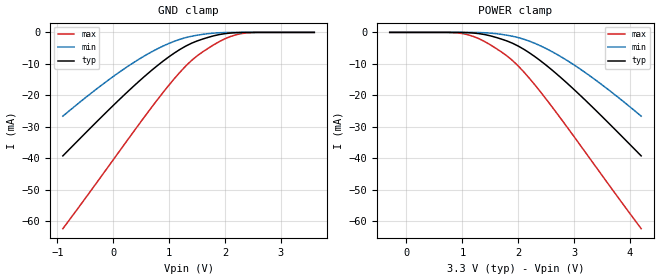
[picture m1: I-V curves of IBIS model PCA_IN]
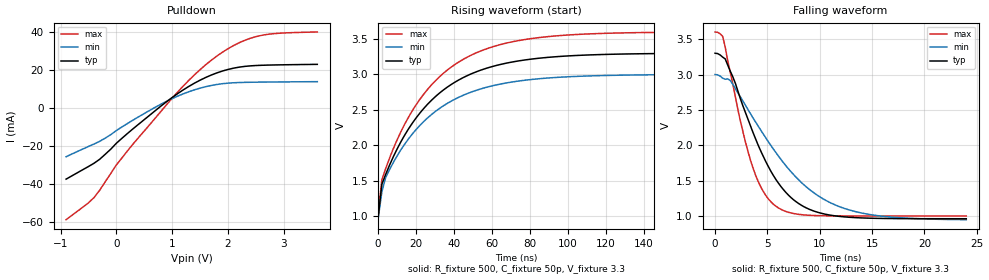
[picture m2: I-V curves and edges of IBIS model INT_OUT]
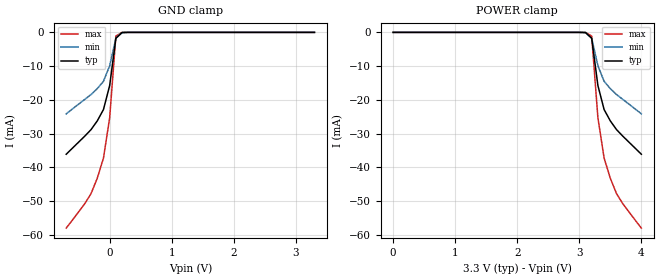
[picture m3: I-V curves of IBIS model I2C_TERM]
|  PCA9541 IBIS MODEL  by NXP Semiconductors, Specialty Logic, Tempe, AZ
|  2-to-1 I2C demultiplexer with interrupt logic and reset
|   Packages: SO16. TSSOP16, HVQFN16
[IBIS Ver]   3.2
[Comment Char]   |_char
| VDD Typ:3.3V, Min:3v, Max: 3.6v
[File name]   pca9541_3_3v.ibs
[File Rev]   1.0
[Date]   Apr 11, 2008 11:44:40 AM
[Source]
Generated by Seshadri Venkataramanan using IbisToolKit.
[Notes]
[Disclaimer]
(C) Copyright 2007 NXP Semiconductors
All rights reserved
NXP Semiconductors (NXP) does not warrant that this model and any other
accompanying information (Model) accurately or fully represents the
operating characteristics and specifications of the semiconductor
products to which the Model relates.  Moreover, the Model is furnished
on an "as is" and with "all faults" basis, and without support or
warranty of any kind.  NXP disclaims all warranties, whether expressed
or implied or statutory, including without limitation all implied
warranties of non-infringement, merchantability and fitness for any
purpose, and those arising from a course of dealing or usage of trade.
NXP does not convey any license under its or any third party's patents,
copyrights or other intellectual property or proprietary rights.
You and your company assume any and all risks and liability arising out
of the application or use of the Model.
In no event shall NXP be liable for any direct, indirect, special,
consequential or incidental damages, however caused, whether in
warranty, contract or tort (including negligence), strict liability or
other legal theory, including, without limitation, for lost profits,
business interruption, or corruption or loss of data or information,
arising out of or in connection with the use of or the inability to use
the Model, even if NXP has been advised of the possibility of such
damages.
NXP provides the Model as a courtesy to our customers. You and your
company shall not distribute, convey, sell, or give the Model to anyone
else without receiving prior written permission from NXP.
NXP reserves the right to make changes without notice to the Model to
improve reliability, function, or design.
Please be aware that your receipt and subsequent use of the Model shall
serve as acceptance of these terms and conditions.  If you do not
accept these terms, return or destroy the Model immediately.
[Copyright]
2008
[Component]   pca9541-1D
Si_location Pin
Timing_location Pin
[Manufacturer]   NXP Semiconductors
| [Package]   SO16
| [Package]   SO16
[Package]
|  variable   typ   min   max
R_pkg   1.75E-01   1.28E-01   2.11E-01
L_pkg   5.03E-09   3.94E-09   6.26E-09
C_pkg   0.794E-12   0.715E-12   0.869E-12
[Pin] signal_name   model_name   R_pin   L_pin   C_pin
1   INT0B   INT_OUT   1.99E-01  6.26E-09  0.822E-12
2   SDA_MST0   I2C_TERM   2.11E-01  5.46E-09  0.869E-12
3   SCL_MST0   I2C_TERM   1.56E-01  4.44E-09  0.760E-12
4   RESETB   PCA_IN   1.28E-01  3.94E-09  0.717E-12
5   SCL_MST1   I2C_TERM   1.28E-01  3.94E-09  0.715E-12
6   SDA_MST1   I2C_TERM   1.56E-01  4.44E-09  0.760E-12
7   INT1B   INT_OUT   2.11E-01  5.46E-09  0.869E-12
8   VSS   GND   1.99E-01  6.26E-09  0.843E-12
9   A0   PCA_IN   1.99E-01  6.26E-09  0.843E-12
10   A1   PCA_IN   2.11E-01  5.46E-09  0.869E-12
11   A2   PCA_IN   1.56E-01  4.44E-09  0.760E-12
12   A0(I2C_SEL)   PCA_IN   1.28E-01  3.94E-09  0.717E-12
13   SCL_SLAVE   I2C_TERM   1.28E-01  3.94E-09  0.715E-12
14   SDA_SLAVE   I2C_TERM   1.56E-01  4.44E-09  0.760E-12
15   INT_INB   PCA_IN   2.11E-01  5.46E-09  0.869E-12
16   VDD   POWER   1.99E-01  6.26E-09  0.843E-12
[Series Pin Mapping] pin_2 model_name   function_table_group
2   14   PCA_SW1   1
6   14   PCA_SW1   2
3   13   PCA_SW1   1
5   13   PCA_SW1   2
[Series Switch Groups]
|  1 /
On 1 /
|  2/
On 2 /
[Component]   pca9541-1PW
Si_location Pin
Timing_location Pin
[Manufacturer]   NXP Semiconductors
| [Package]   TSSOP16
| [Package]   TSSOP16
[Package]
| variable   typ   min   max
R_pkg   3.95E-02   3.52E-02   4.56E-02
L_pkg   1.94E-09   1.65E-09   2.40E-09
C_pkg   0.446E-12   0.335E-12   0.771E-12
[Pin] signal_name   model_name   R_pin   L_pin   C_pin
1   INT0B   INT_OUT   3.52E-02  2.40E-09  0.436E-12
2   SDA_MST0   I2C_TERM   3.70E-02  1.93E-09  0.438E-12
3   SCL_MST0   I2C_TERM   4.56E-02  1.76E-09  0.345E-12
4   RESETB   PCA_IN   4.00E-02  1.65E-09  0.335E-12
5   SCL_MST1   I2C_TERM   4.00E-02  1.65E-09  0.335E-12
6   SDA_MST1   I2C_TERM   4.56E-02  1.76E-09  0.345E-12
7   INT1B   INT_OUT   3.70E-02  1.93E-09  0.438E-12
8   VSS   GND   3.52E-02  2.40E-09  0.452E-12
9   A0   PCA_IN   3.52E-02  2.40E-09  0.452E-12
10   A1   PCA_IN   3.70E-02  1.93E-09  0.438E-12
11   A2   PCA_IN   4.56E-02  1.76E-09  0.345E-12
12   A0(I2C_SEL)   PCA_IN   4.00E-02  1.65E-09  0.771E-12
13   SCL_SLAVE   I2C_TERM   4.00E-02  1.65E-09  0.771E-12
14   SDA_SLAVE   I2C_TERM   4.56E-02  1.76E-09  0.345E-12
15   INT_INB   PCA_IN   3.70E-02  1.93E-09  0.438E-12
16   VDD   POWER   3.52E-02  2.40E-09  0.452E-12
[Series Pin Mapping] pin_2 model_name   function_table_group
2   14   PCA_SW1   1
6   14   PCA_SW1   2
3   13   PCA_SW1   1
5   13   PCA_SW1   2
[Series Switch Groups]
|  1 /
On 1 /
|  2/
On 2 /
[Component]   pca9541-1BS
Si_location Pin
Timing_location Pin
[Manufacturer]   NXP Semiconductors
[Package]
|  variable   typ   min   max
R_pkg   403m   325m   479m
L_pkg   112nh   98nh   127nh
C_pkg   0.142p   0.129p   0.157p
[Package Model]   hvqfn16
[Pin] signal_name   model_name
1   SCL_MST0   I2C_TERM
2   RESETB   PCA_IN
3   SCL_MST1   I2C_TERM
4   SDA_MST1   I2C_TERM
5   INT1B   INT_OUT
6   VSS   GND
7   A0   PCA_IN
8   A1   PCA_IN
9   A2   PCA_IN
10   A0(I2C_SEL)   PCA_IN
11   SCL_SLAVE   I2C_TERM
12   SDA_SLAVE   I2C_TERM
13   INT_INB   PCA_IN
14   VDD   POWER
15   INT0B   INT_OUT
16   SDA_MST0   I2C_TERM
[Series Pin Mapping] pin_2 model_name   function_table_group
16   12   PCA_SW1   1
4   12   PCA_SW1   2
1   11   PCA_SW1   1
3   11   PCA_SW1   2
[Series Switch Groups]
|  1 /
On 1 /
|  2/
On 2 /
[Define Package Model]   hvqfn16
[Manufacturer]   Unknown
[OEM]   Unknown
[Description]   none
[Number of Pins]   16
[Pin Numbers]
|   1 =
1
|   2 =
2
|   3 =
3
|   4 =
4
|   5 =
5
|   6 =
6
|   7 =
7
|   8 =
8
|   9 =
9
|   10 =
10
|   11 =
11
|   12 =
12
|   13 =
13
|   14 =
14
|   15 =
15
|   16 =
16
[Model Data]
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[End Model Data]
[End Package Model]
[Model]   PCA_SW1
Model_type Series_switch
C_comp   5.5p   5.3p   5.7p
[Temperature Range] 27   85   -40
[Voltage Range]   3.3   3   3.6
[On]
[R Series]   12   4   24
[L Series]   0   0   0
[C Series]   2p   1p   5p
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[Off]
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| Models and submodels in the file (4): PCA_IN (Input), INT_OUT (Open_drain), I2C_TERM (Terminator), PCA_SW1 (Series_switch)
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[Model]   PCA_IN
Model_type Input
Vinh=2.1
Vinl=0.9
C_comp   2.44p   2.2p   2.6p
[Temperature Range] 27   85   -40
[Voltage Range]   3.3   3   3.6
[GND Clamp]
-900mV    -39.22mA   -26.6mA    -62.33mA
-100mV    -24.97mA   -15.33mA   -42.96mA
500mV     -14.94mA   -8.108mA   -28.28mA
800mV     -10.43mA   -5.142mA   -21.2mA
1.1V      -6.496mA   -2.786mA   -14.59mA
1.3V      -4.347mA   -1.651mA   -10.68mA
1.5V      -2.735mA   -904.6uA   -7.49mA
1.9V      -688.8uA   -114uA     -2.915mA
2.1V      -205uA     -16.81uA   -1.301mA
2.3V      -30.06uA   -1.317uA   -370uA
2.6V      -376.8nA   -17.96nA   -10.03uA
3.6V      11.35pA    121.4pA    -358.3fA
[POWER Clamp]
-300mV    11.35pA    121.4pA    -358.3fA
700mV     -376.8nA   -17.96nA   -10.03uA
1V        -30.06uA   -1.317uA   -370uA
1.2V      -205uA     -16.81uA   -1.301mA
1.4V      -688.8uA   -114uA     -2.915mA
1.8V      -2.735mA   -904.6uA   -7.49mA
2V        -4.347mA   -1.651mA   -10.68mA
2.2V      -6.496mA   -2.786mA   -14.59mA
2.5V      -10.43mA   -5.142mA   -21.2mA
2.8V      -14.94mA   -8.108mA   -28.28mA
3.4V      -24.97mA   -15.33mA   -42.96mA
4.2V      -39.22mA   -26.6mA    -62.33mA
[Model]   INT_OUT
Model_type Open_drain
Vref=3.3
Vmeas=1.65
Rref=1000
Cref=50p
C_comp   2.44p   2.2p   2.6p
[Model Spec]
Vmeas   1.65   1.485   1.815
[Temperature Range] 27   85   -40
[Voltage Range]   3.3   3   3.6
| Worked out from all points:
|   slope of the pulldown table from 0 to 0.495 V, typ, clamps not added: 40.1 ohm
|   falling waveform, R_fixture 500, C_fixture 50p, V_fixture 3.3: 20-80 % time 4.2ns typ, 6.36ns min, 2.65ns max; typ from 3.3 V to 0.966 V
|   rising waveform, R_fixture 500, C_fixture 50p, V_fixture 3.3: 20-80 % time 35.2ns typ, 34.2ns min, 35.2ns max; typ from 0.966 V to 3.3 V
[Pulldown]
-900mV    -37.63mA   -25.83mA   -59mA
-400mV    -29.27mA   -19.11mA   -47.35mA
-300mV    -27.2mA    -17.72mA   -43.56mA
0V        -18.73mA   -12.01mA   -30.14mA
600mV     -3.874mA   -1.355mA   -8.841mA
1V        5.408mA    4.822mA    5.042mA
1.4V      12.97mA    9.452mA    17.37mA
1.8V      18.37mA    12.27mA    27.24mA
2.2V      21.41mA    13.3mA     34.26mA
2.5V      22.26mA    13.48mA    37.48mA
2.9V      22.6mA     13.6mA     39.25mA
3.6V      22.88mA    13.76mA    39.95mA
[Falling Waveform]
R_fixture=500
C_fixture=50p
V_fixture=3.3
V_fixture_min=3
V_fixture_max=3.6
0s        3.3V       3V         3.6V
727.3ps   3.245V     2.948V     3.539V
1.455ns   3.046V     2.915V     3.031V
2.424ns   2.656V     2.684V     2.342V
3.636ns   2.178V     2.385V     1.677V
4.606ns   1.846V     2.161V     1.351V
5.818ns   1.518V     1.898V     1.143V
8.485ns   1.136V     1.445V     1.02V
12.36ns   992mV      1.111V     1.005V
24ns      965.8mV    952.6mV    1.004V
[Rising Waveform]
R_fixture=500
C_fixture=50p
V_fixture=3.3
V_fixture_min=3
V_fixture_max=3.6
0s        965.7mV    948.4mV    1.004V
2.02ns    1.448V     1.34V      1.512V
4.04ns    1.589V     1.545V     1.671V
6.061ns   1.718V     1.655V     1.818V
16.16ns   2.236V     2.094V     2.402V
30.3ns    2.69V      2.48V      2.914V
48.48ns   3.002V     2.745V     3.265V
68.69ns   3.166V     2.885V     3.45V
94.95ns   3.253V     2.96V      3.548V
200ns     3.3V       3V         3.6V
[Ramp]
R_load=500
dV/dt_r   1.399E+0/1.893E-9   1.385E+0/1.815E-9   1.383E+0/1.077E-9
dV/dt_f   1.401E+0/3.280E-10   1.388E+0/1.160E-9   1.387E+0/3.385E-10
|[End   INT_OUT
| [End   SDAX,SCLX
[Model]   I2C_TERM
Model_type Terminator
C_comp   5.5p   5.3p   5.7p
[Temperature Range] 27   85   -40
[Voltage Range]   3.3   3   3.6
[GND Clamp]
-700mV    -36.14mA   -24.16mA   -58.06mA
-400mV    -30.75mA   -19.86mA   -50.77mA
-300mV    -28.84mA   -18.43mA   -47.81mA
-200mV    -26.25mA   -16.69mA   -43.25mA
-100mV    -22.88mA   -14.5mA    -37.28mA
0V        -15.76mA   -9.893mA   -25.32mA
100mV     -1.746mA   -1.727mA   -1.088mA
200mV     -44.67uA   -89.07uA   -8.197uA
3.3V      204.9pA    234.9pA    202.8pA
[POWER Clamp]
0V        204.9pA    234.9pA    202.8pA
3.1V      -44.67uA   -89.07uA   -8.197uA
3.2V      -1.746mA   -1.727mA   -1.088mA
3.3V      -15.76mA   -9.893mA   -25.32mA
3.4V      -22.88mA   -14.5mA    -37.28mA
3.5V      -26.25mA   -16.69mA   -43.25mA
3.6V      -28.84mA   -18.43mA   -47.81mA
3.7V      -30.75mA   -19.86mA   -50.77mA
4V        -36.14mA   -24.16mA   -58.06mA
